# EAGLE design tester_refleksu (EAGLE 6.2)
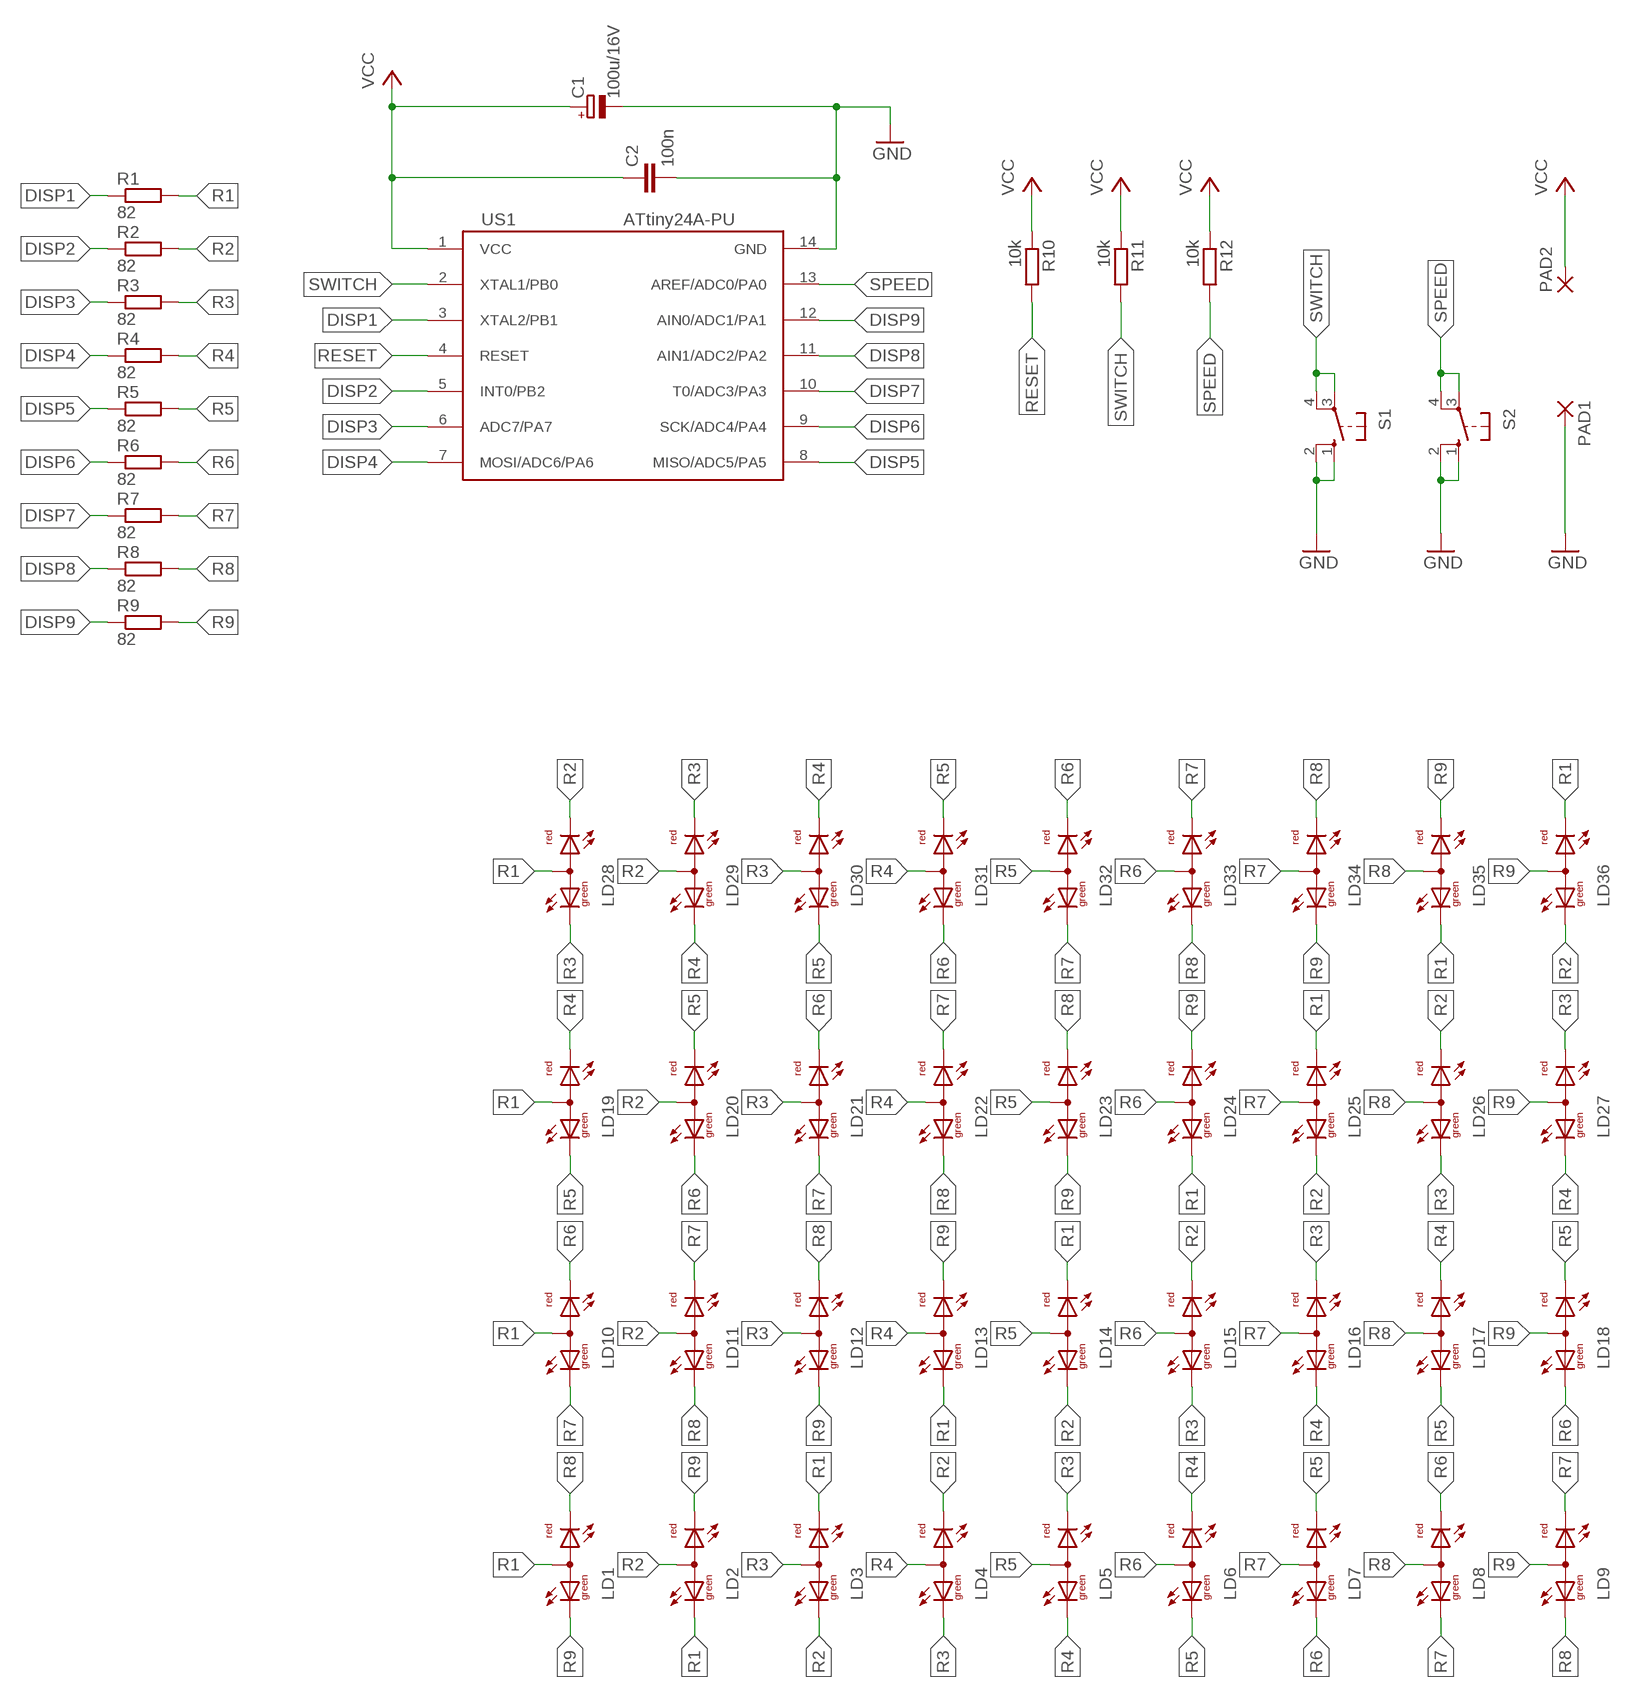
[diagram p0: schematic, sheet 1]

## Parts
C1  100u/16V  CPOL-EUTT2D5L  [TT2D5L]
C2  100n  C-EU050-025X075  [C050-025X075]
LD1  DUOLED-RG-A  [DUOLED-A-5MM]
LD2  DUOLED-RG-A  [DUOLED-A-5MM]
LD3  DUOLED-RG-A  [DUOLED-A-5MM]
LD4  DUOLED-RG-A  [DUOLED-A-5MM]
LD5  DUOLED-RG-A  [DUOLED-A-5MM]
LD6  DUOLED-RG-A  [DUOLED-A-5MM]
LD7  DUOLED-RG-A  [DUOLED-A-5MM]
LD8  DUOLED-RG-A  [DUOLED-A-5MM]
LD9  DUOLED-RG-A  [DUOLED-A-5MM]
LD10  DUOLED-RG-A  [DUOLED-A-5MM]
LD11  DUOLED-RG-A  [DUOLED-A-5MM]
LD12  DUOLED-RG-A  [DUOLED-A-5MM]
LD13  DUOLED-RG-A  [DUOLED-A-5MM]
LD14  DUOLED-RG-A  [DUOLED-A-5MM]
LD15  DUOLED-RG-A  [DUOLED-A-5MM]
LD16  DUOLED-RG-A  [DUOLED-A-5MM]
LD17  DUOLED-RG-A  [DUOLED-A-5MM]
LD18  DUOLED-RG-A  [DUOLED-A-5MM]
LD19  DUOLED-RG-A  [DUOLED-A-5MM]
LD20  DUOLED-RG-A  [DUOLED-A-5MM]
LD21  DUOLED-RG-A  [DUOLED-A-5MM]
LD22  DUOLED-RG-A  [DUOLED-A-5MM]
LD23  DUOLED-RG-A  [DUOLED-A-5MM]
LD24  DUOLED-RG-A  [DUOLED-A-5MM]
LD25  DUOLED-RG-A  [DUOLED-A-5MM]
LD26  DUOLED-RG-A  [DUOLED-A-5MM]
LD27  DUOLED-RG-A  [DUOLED-A-5MM]
LD28  DUOLED-RG-A  [DUOLED-A-5MM]
LD29  DUOLED-RG-A  [DUOLED-A-5MM]
LD30  DUOLED-RG-A  [DUOLED-A-5MM]
LD31  DUOLED-RG-A  [DUOLED-A-5MM]
LD32  DUOLED-RG-A  [DUOLED-A-5MM]
LD33  DUOLED-RG-A  [DUOLED-A-5MM]
LD34  DUOLED-RG-A  [DUOLED-A-5MM]
LD35  DUOLED-RG-A  [DUOLED-A-5MM]
LD36  DUOLED-RG-A  [DUOLED-A-5MM]
PAD1  3,17/1,3  [3,17/1,3]
PAD2  3,17/1,3  [3,17/1,3]
R1  82  R-EU_0207/7  [0207/7]
R2  82  R-EU_0207/7  [0207/7]
R3  82  R-EU_0207/7  [0207/7]
R4  82  R-EU_0207/7  [0207/7]
R5  82  R-EU_0207/7  [0207/7]
R6  82  R-EU_0207/7  [0207/7]
R7  82  R-EU_0207/7  [0207/7]
R8  82  R-EU_0207/7  [0207/7]
R9  82  R-EU_0207/7  [0207/7]
R10  10k  R-EU_0207/7  [0207/7]
R11  10k  R-EU_0207/7  [0207/7]
R12  10k  R-EU_0207/7  [0207/7]
S1  40-XX  [B3F-40XX]
S2  10-XX  [B3F-10XX]
US1  ATtiny24A-PU  ATTINY24/44/84-PU  [DIL14]

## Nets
DISP1: R1.1 US1.3(XTAL2/PB1)
DISP2: R2.1 US1.5(INT0/PB2)
DISP3: R3.1 US1.6(ADC7/PA7)
DISP4: R4.1 US1.7(MOSI/ADC6/PA6)
DISP5: R5.1 US1.8(MISO/ADC5/PA5)
DISP6: R6.1 US1.9(SCK/ADC4/PA4)
DISP7: R7.1 US1.10(T0/ADC3/PA3)
DISP8: R8.1 US1.11(AIN1/ADC2/PA2)
DISP9: R9.1 US1.12(AIN0/ADC1/PA1)
GND: C1.- C2.2 PAD1.1(P) S1.1(S) S1.2(S1) S2.1(S) S2.2(S1) US1.14(GND)
R1: LD1.A LD2.CX(CG) LD3.CR LD10.A LD13.CX(CG) LD14.CR LD19.A LD24.CX(CG) LD25.CR LD28.A LD35.CX(CG) LD36.CR R1.2
R2: LD2.A LD3.CX(CG) LD4.CR LD11.A LD14.CX(CG) LD15.CR LD20.A LD25.CX(CG) LD26.CR LD28.CR LD29.A LD36.CX(CG) R2.2
R3: LD3.A LD4.CX(CG) LD5.CR LD12.A LD15.CX(CG) LD16.CR LD21.A LD26.CX(CG) LD27.CR LD28.CX(CG) LD29.CR LD30.A R3.2
R4: LD4.A LD5.CX(CG) LD6.CR LD13.A LD16.CX(CG) LD17.CR LD19.CR LD22.A LD27.CX(CG) LD29.CX(CG) LD30.CR LD31.A R4.2
R5: LD5.A LD6.CX(CG) LD7.CR LD14.A LD17.CX(CG) LD18.CR LD19.CX(CG) LD20.CR LD23.A LD30.CX(CG) LD31.CR LD32.A R5.2
R6: LD6.A LD7.CX(CG) LD8.CR LD10.CR LD15.A LD18.CX(CG) LD20.CX(CG) LD21.CR LD24.A LD31.CX(CG) LD32.CR LD33.A R6.2
R7: LD7.A LD8.CX(CG) LD9.CR LD10.CX(CG) LD11.CR LD16.A LD21.CX(CG) LD22.CR LD25.A LD32.CX(CG) LD33.CR LD34.A R7.2
R8: LD1.CR LD8.A LD9.CX(CG) LD11.CX(CG) LD12.CR LD17.A LD22.CX(CG) LD23.CR LD26.A LD33.CX(CG) LD34.CR LD35.A R8.2
R9: LD1.CX(CG) LD2.CR LD9.A LD12.CX(CG) LD13.CR LD18.A LD23.CX(CG) LD24.CR LD27.A LD34.CX(CG) LD35.CR LD36.A R9.2
RESET: R10.2 US1.4(RESET)
SPEED: R12.2 S2.3(P) S2.4(P1) US1.13(AREF/ADC0/PA0)
SWITCH: R11.2 S1.3(P) S1.4(P1) US1.2(XTAL1/PB0)
VCC: C1.+ C2.1 PAD2.1(P) R10.1 R11.1 R12.1 US1.1(VCC)

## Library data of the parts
C1 = rcl:CPOL-EU: POLARIZED CAPACITOR, European symbol
C2 = rcl:C-EU: CAPACITOR, European symbol
LD1-LD36 = led:DUOLED-RG-A: DUO LED 2 colors (red/green), 3mm or 5mm, round, common Anode
PAD1 PAD2 = wirepad:3,17/1,3: THROUGH-HOLE PAD
R1-R12 = rcl:R-EU_: RESISTOR, European symbol
S1 = switch-omron:40-XX: OMRON SWITCH; MF: OMRON COMPONENTS USA; MPN: B3F-4000; OC_FARNELL: 176434; OC_NEWARK: 36K3105
S2 = switch-omron:10-XX: OMRON SWITCH; MPN: B3F-1000; OC_FARNELL: 176432; OC_NEWARK: 36M3542
US1 = scalaki_futrzak:ATTINY24/44/84

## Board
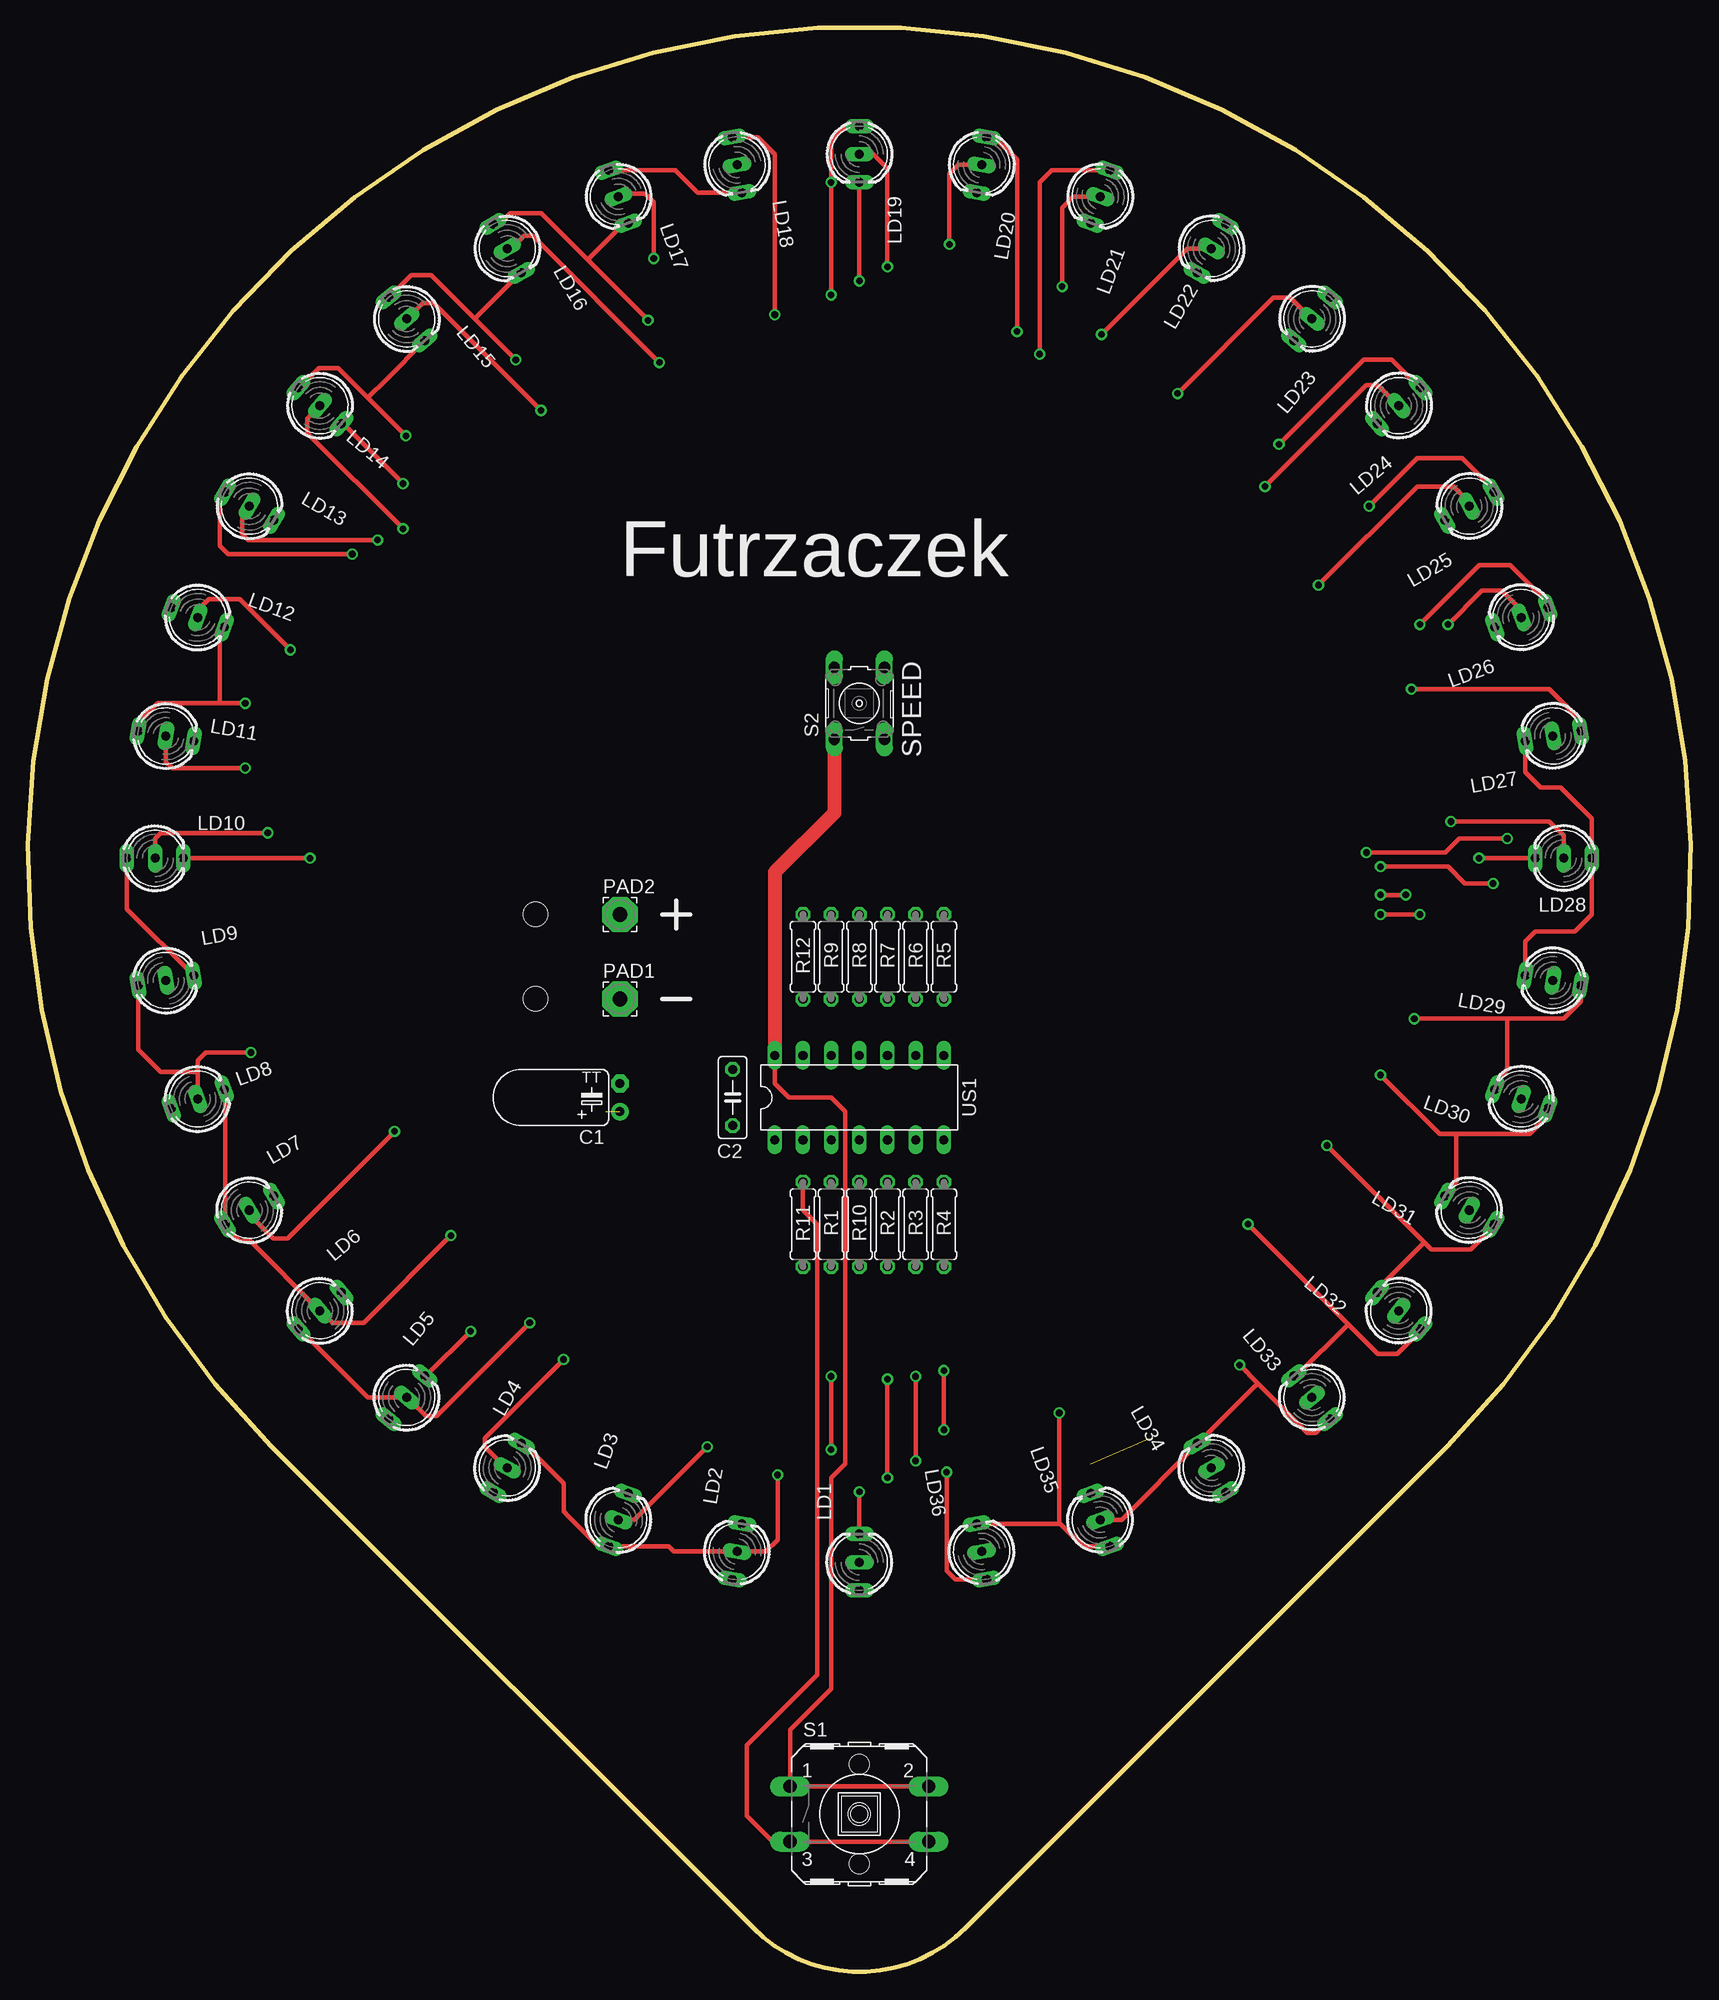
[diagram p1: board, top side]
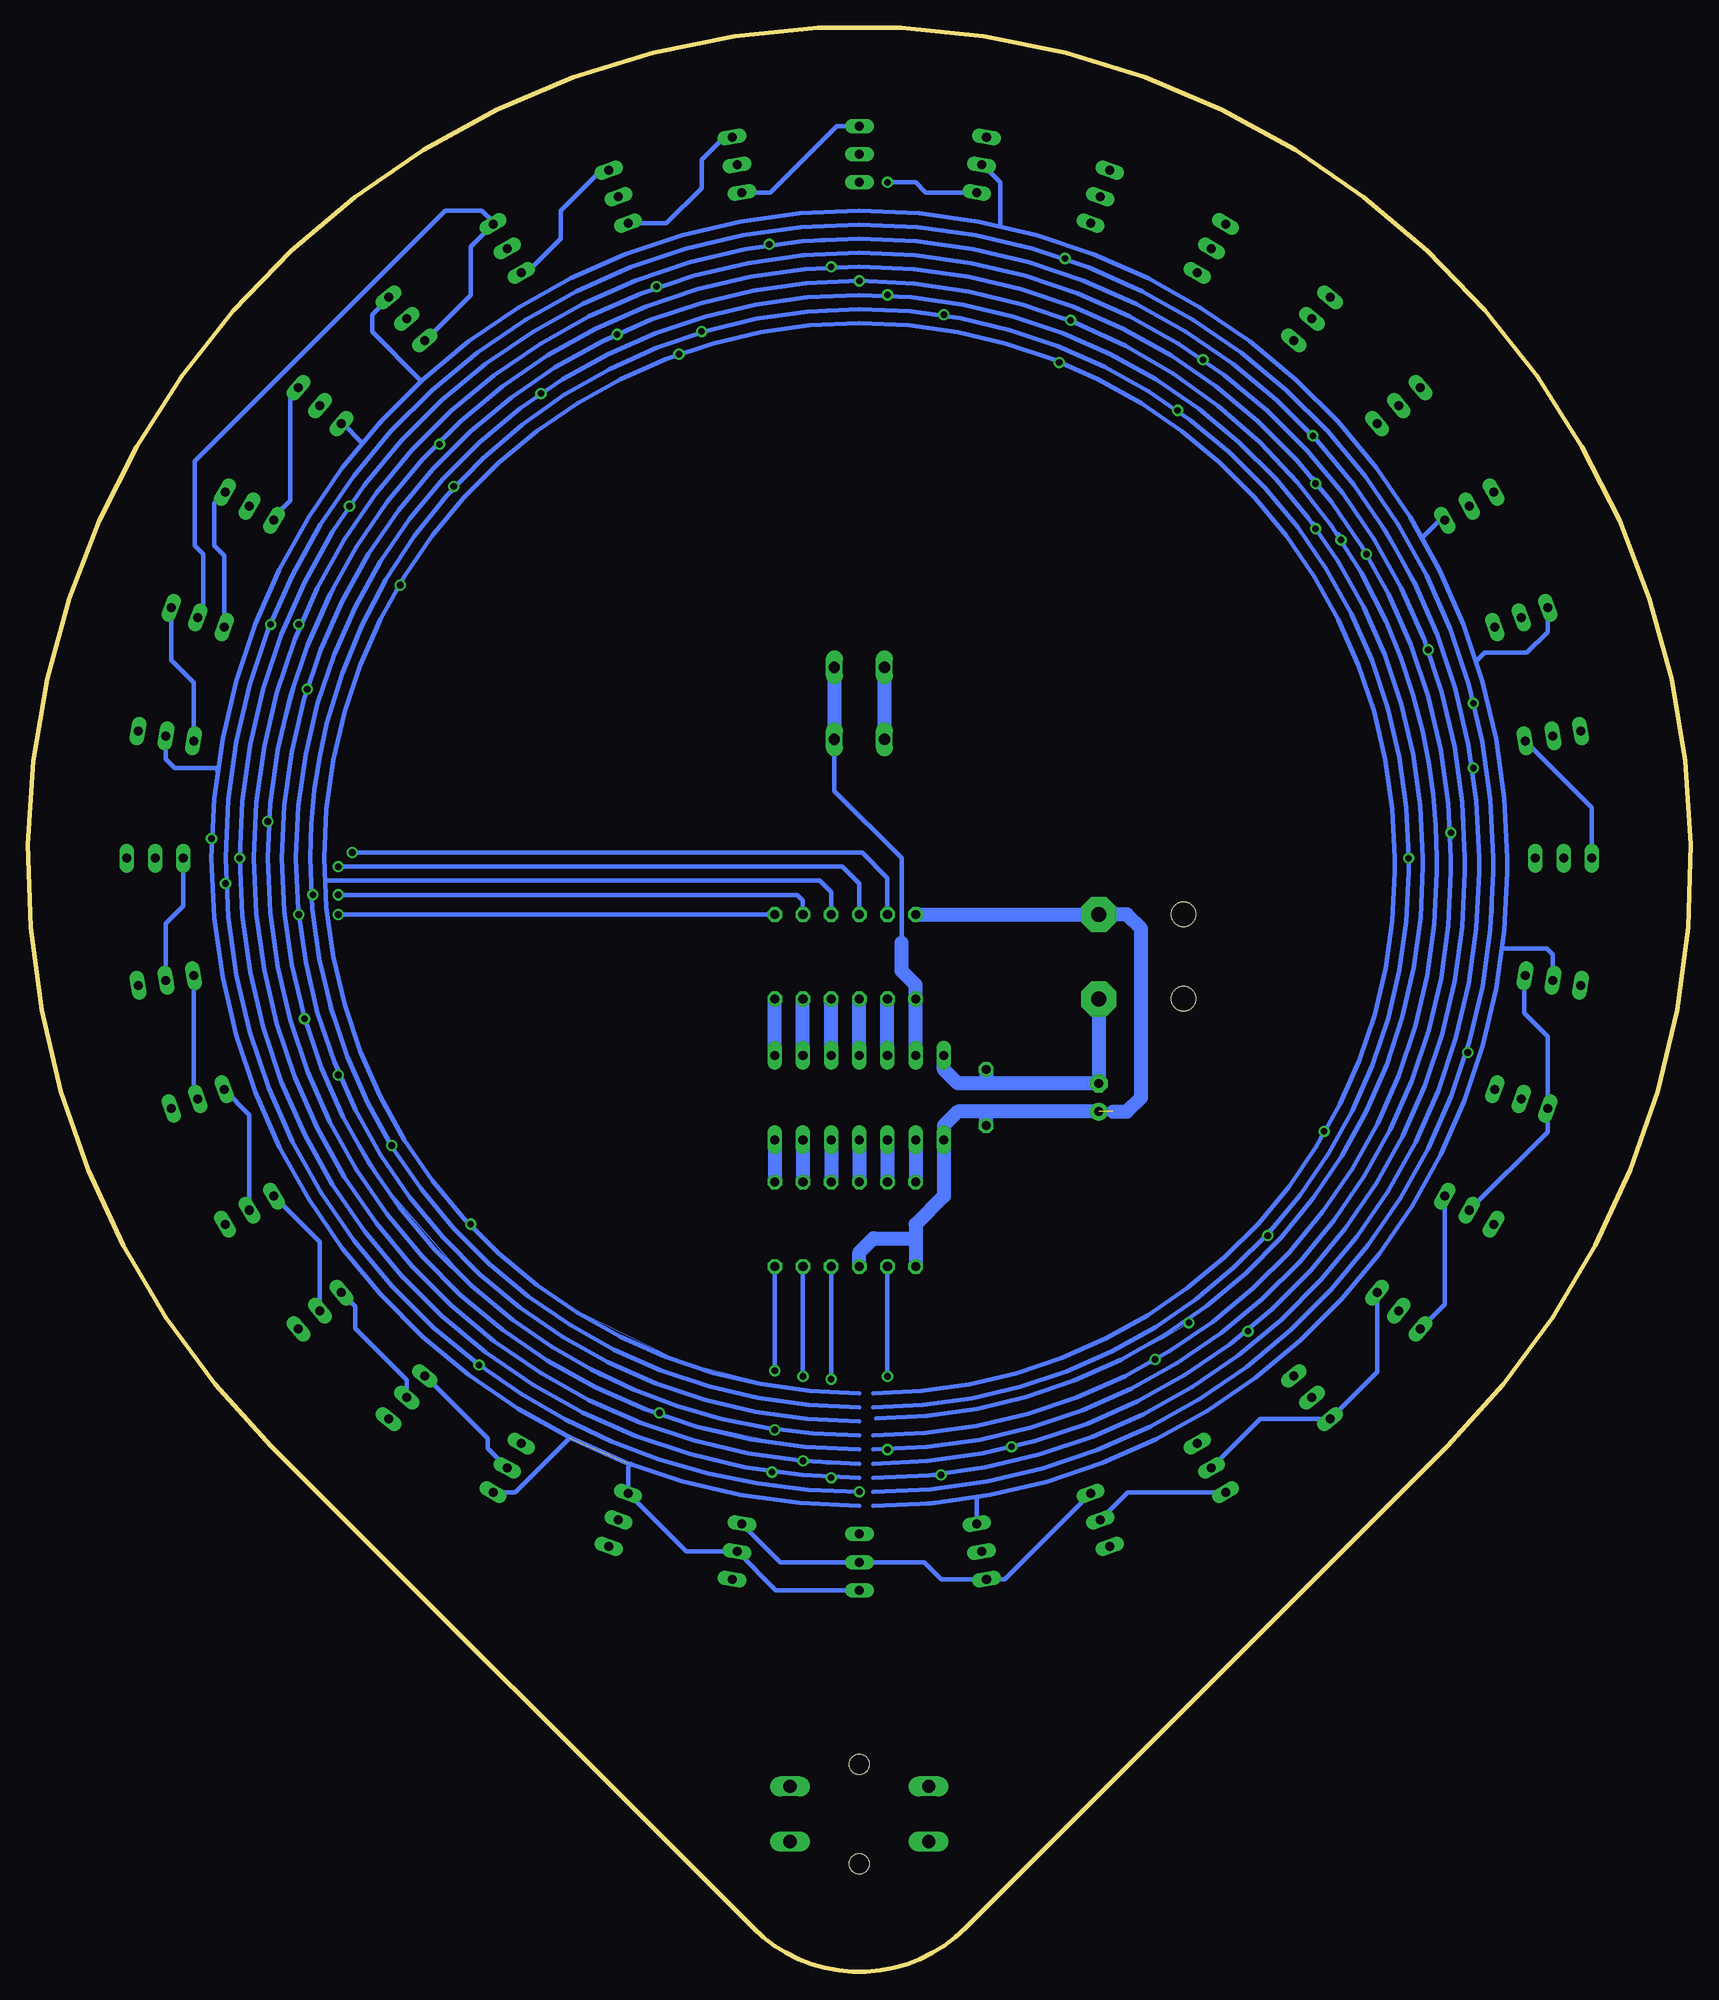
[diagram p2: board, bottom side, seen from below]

Size 149.98 x 175.35 mm. Coordinates in mm from the lower left corner, seen from the top.
Outline: 21.96,47.41 65.42,3.95 arc90 84.56,3.95 128.02,47.41 arc270 21.96,47.41
Copper layers (1*16): Top 0.035mm / dielectric 1.5mm / Bottom 0.035mm
Design rules: minimum track width 10mil, minimum drill 23mil, track to track 8mil, track to pad 8mil, pad to pad 8mil, via to via 8mil, smd to smd 8mil, copper to edge 15mil, drill to drill 8mil, minimum pad ring 10mil, minimum via ring 8mil, stop-mask expansion 4mil, vias tented up to drill 0mil, thermal gap 10mil
Holes 2.2 mm at 45.78,87.74 45.78,95.36

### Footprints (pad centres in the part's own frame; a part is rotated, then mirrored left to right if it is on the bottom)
TT2D5L = drill 0.813 pad 1.6: + -1.27,0 | drill 0.813 pad 1.6 octagon: - 1.27,0
C050-025X075 = drill 0.813 octagon: 1 -2.54,0; 2 2.54,0
DUOLED-A-5MM = drill 0.813 long: A 0,0; CR 2.54,0; CX -2.54,0
3,17/1,3 = drill 1.321 pad 3.175 octagon: 1 0,0
0207/7 = drill 0.813 octagon: 1 -3.81,0; 2 3.81,0
B3F-40XX = drill 1.194 long: 1 -6.248,2.489; 2 6.248,2.489; 3 -6.248,-2.489; 4 6.248,-2.489 | hole 1.803: 0,-4.496; 0,4.496
B3F-10XX = drill 1.016 long: 1 -3.251,2.261; 2 3.251,2.261; 3 -3.251,-2.261; 4 3.251,-2.261
DIL14 = drill 0.813 long: 1 -7.62,-3.81; 2 -5.08,-3.81; 3 -2.54,-3.81; 4 0,-3.81; 5 2.54,-3.81; 6 5.08,-3.81; 7 7.62,-3.81; 8 7.62,3.81; 9 5.08,3.81; 10 2.54,3.81; 11 0,3.81; 12 -2.54,3.81; 13 -5.08,3.81; 14 -7.62,3.81

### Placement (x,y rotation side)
C1  53.4,78.85 90 top
C2  63.56,78.85 90 top
LD1  74.99,36.94 90 top
LD2  63.96,37.91 80 top
LD3  53.27,40.77 70 top
LD4  43.24,45.45 60 top
LD5  34.17,51.8 50 top
LD6  26.35,59.63 40 top
LD7  20,68.69 30 top
LD8  15.32,78.72 20 top
LD9  12.45,89.42 10 top
LD10  11.49,100.44 0 top
LD11  12.45,111.47 350 top
LD12  15.32,122.16 340 top
LD13  20,132.19 330 top
LD14  26.35,141.26 320 top
LD15  34.17,149.09 310 top
LD16  43.24,155.44 300 top
LD17  53.27,160.11 290 top
LD18  63.96,162.98 280 top
LD19  74.99,163.94 270 top
LD20  86.02,162.98 260 top
LD21  96.71,160.11 250 top
LD22  106.74,155.44 240 top
LD23  115.81,149.09 230 top
LD24  123.63,141.26 220 top
LD25  129.98,132.19 210 top
LD26  134.66,122.16 200 top
LD27  137.52,111.47 190 top
LD28  138.49,100.44 180 top
LD29  137.52,89.42 170 top
LD30  134.66,78.72 160 top
LD31  129.98,68.69 150 top
LD32  123.63,59.63 140 top
LD33  115.81,51.8 130 top
LD34  106.74,45.45 120 top
LD35  96.71,40.77 110 top
LD36  86.02,37.91 100 top
PAD1  53.4,87.74 0 top
PAD2  53.4,95.36 0 top
R1  72.45,67.42 270 top
R2  77.53,67.42 270 top
R3  80.07,67.42 270 top
R4  82.61,67.42 270 top
R5  82.61,91.55 90 top
R6  80.07,91.55 90 top
R7  77.53,91.55 90 top
R8  74.99,91.55 90 top
R9  72.45,91.55 90 top
R10  74.99,67.42 90 top
R11  69.91,67.42 90 top
R12  69.91,91.55 270 top
S1  74.99,14.23 0 top
S2  74.99,114.41 90 top
US1  74.99,78.85 0 top

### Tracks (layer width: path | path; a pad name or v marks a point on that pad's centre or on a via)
DISP1
  Bottom 1.27: US1.3 R1.1
DISP2
  Bottom 1.27: US1.5 R2.1
DISP3
  Bottom 1.27: US1.6 R3.1
DISP4
  Bottom 1.27: US1.7 R4.1
DISP5
  Bottom 1.27: US1.8 R5.1
DISP6
  Bottom 1.27: US1.9 R6.1
DISP7
  Bottom 1.27: US1.10 R7.1
DISP8
  Bottom 1.27: US1.11 R8.1
DISP9
  Bottom 1.27: US1.12 R9.1
GND
  Top 0.406: S1.2 S1.1 68.74,21.81 72.45,25.51 72.45,44.56 73.72,45.83 73.72,77.58 72.45,78.85 68.64,78.85 67.37,80.12 US1.14
  Top 1.27: S2.1 72.73,104.53 67.37,99.17 US1.14
  Bottom 1.27: 63.56,80.12 C1.- PAD1.1 | 63.56,80.12 66.1,80.12 67.37,81.39 US1.14 | C2.2 63.56,80.12 | S2.2 S2.1
R1  (via drill 0.6)
  Top 0.406: LD19.A 76.26,163.94 77.53,162.67 v77.53,153.78 | LD24.CX 125.5,142.89 123,145.4 120.46,145.4 v112.84,137.78 | LD28.A 138.49,102.48 137.22,103.75 v128.33,103.75 | LD35.CX 95.14,38.39 94.29,39.23 93.02,40.5 | 93.02,40.5 v93.02,50.41 | LD36.CR 92.93,40.41 93.02,40.5 | LD10.A 11.49,102.22 12,102.73 v21.65,102.73 | LD13.CX 17.8,133.17 17.33,132.7 17.33,128.64 18.09,127.88 v29.27,127.88 | LD14.CR 28.44,139.63 v33.84,134.23 | v72.45,53.71 v72.45,47.1
  Bottom 0: 128.33,100.44 v128.33,103.75 128.08,106.03 127.57,109.33 125.28,117.97 120.96,127.62 115.63,134.99 v112.84,137.78 | 74.99,47.1 78.55,47.1 83.12,47.87 89.98,49.39 v93.02,50.41 | 73.72,47.1 v72.45,47.1 | 21.65,100.44 v21.65,102.73 21.9,106.29 22.41,109.08 22.67,111.37 24.19,116.95 24.95,118.99 25.97,121.27 26.73,123.3 v29.27,127.88 | 29.52,128.13 33.08,133.46 v33.84,134.23 | v77.53,153.78 74.99,153.78
  Bottom 0.406: 74.99,47.1 arc90 128.33,100.44 arc90 74.99,153.78 arc90 21.65,100.44 21.65,99.17 arc90 73.72,47.1 | LD25.CR 127.78,131.22 126.3,132.7 126.3,142.17 LD24.CX | LD36.CR 82.11,36.94 LD1.A 69.15,36.94 67.61,35.41 LD2.CX 61.89,35.41 LD3.CR | v21.65,102.73 21.65,102.22 | v29.27,127.88 29.52,128.13 | v33.84,134.23 33.84,134.48 34.1,134.73 | R1.2 v72.45,53.71 | v72.45,47.1 72.2,47.1
R2  (via drill 0.6)
  Top 0.406: LD20.A 83.93,162.98 83.12,162.17 v83.12,155.82 | LD25.CX 132.18,133.68 129.35,136.51 125.28,136.51 v120.96,132.19 | LD28.CR v130.87,100.44 | LD36.CX 83.64,35.41 82.86,36.18 v82.86,45.07 | v67.62,44.82 67.62,38.98 66.56,37.91 LD2.A 58.28,37.91 57.97,38.21 57.8,38.39 LD3.CX 51.45,38.39 48.83,41.01 48.32,41.52 48.32,44.06 44.72,47.65 LD4.CR | LD11.A 12.45,109.13 13.01,108.57 v19.62,108.57 | LD14.CX 24.48,142.89 26.22,144.64 28,144.64 30.67,141.97 | 30.67,141.97 v34.1,138.54 | LD15.CR 35.81,147.11 32.32,143.62 30.67,141.97 | v77.53,53.45 v77.53,44.56
  Bottom 0: v130.87,100.44 130.36,107.3 129.35,113.14 128.58,116.19 127.31,120.26 126.04,123.3 124.01,127.37 v120.96,132.19 | 77.28,44.56 74.99,44.56 | v82.86,45.07 79.31,44.82 v77.53,44.56 | 68.39,44.82 71.18,44.56 73.72,44.56 | 19.11,100.44 19.36,104.76 v19.62,108.57 | 19.87,109.08 20.38,112.89 23.43,122.03 26.48,127.88 28.76,131.69 31.3,135.24 v34.1,138.54 | 74.99,156.32 78.55,156.32 81.34,156.07 v83.12,155.82
  Bottom 0.406: 74.99,44.56 arc90 v130.87,100.44 arc90 74.99,156.32 arc90 19.11,100.44 19.11,99.17 arc90 73.72,44.56 | LD26.CR 132.27,127.76 133.16,128.64 133.16,132.49 LD25.CX | LD28.CR 135.95,96.13 137.52,94.55 LD29.A | v67.62,44.82 68.39,44.82 | v19.62,108.57 19.62,108.83 19.87,109.08 | v34.1,138.54 34.35,138.8 | R2.2 v77.53,53.45 | v77.53,44.56 77.28,44.56
R3  (via drill 0.6)
  Top 0.406: LD21.A 94.27,160.11 93.28,159.12 v93.28,152.01 | LD26.CX 137.05,123.48 133.66,126.86 130.87,126.86 v125.54,121.53 | LD27.CR 135.02,108.23 136.46,106.79 138.24,106.79 141.03,104 LD28.CX 141.03,95.36 139.51,93.84 135.95,93.84 135.02,92.91 LD29.CR | LD3.A 54.69,40.77 v61.27,47.36 | LD5.CR 35.91,53.75 v39.94,57.77 | LD12.A 15.32,122.82 16.32,123.81 19.11,123.81 v23.68,119.24 | LD15.CX 32.62,151.03 34.6,153.02 36.38,153.02 40.32,149.08 | 40.32,149.08 v44,145.4 | LD16.CR 44.47,153.24 40.32,149.08 | v80.07,53.71 v80.07,46.09
  Bottom 0: 129.6,100.44 129.35,105.78 128.58,110.86 126.3,118.99 v125.54,121.53 | 79.82,46.09 78.04,45.83 74.99,45.83 | 73.72,45.83 71.69,45.83 67.37,46.34 62.54,47.1 v61.27,47.36 59.75,47.61 53.15,49.9 47.05,52.95 43.24,55.49 v39.94,57.77 | 20.38,104 20.89,108.57 21.9,112.89 22.67,115.94 v23.68,119.24 22.41,115.18 21.14,110.1 20.38,104 | v93.28,152.01 89.98,153.02 83.88,154.29 79.05,154.8 76.51,155.05 74.99,155.05 73.21,155.05 70.16,154.8 64.32,154.04 60.26,153.02 54.16,150.99 49.59,148.7 45.53,146.42 v44,145.4 | 20.38,104 20.38,100.44
  Bottom 0.406: 74.99,45.83 arc90 129.6,100.44 arc90 74.99,155.05 arc90 20.38,100.44 20.38,99.17 arc90 73.72,45.83 | LD27.CR 135.02,116.28 137.05,118.3 LD26.CX | LD29.CR 135.02,79.09 LD30.A | LD4.CX 50.79,43.25 LD3.A | v23.68,119.24 23.94,119.49 | R3.2 v80.07,53.71 | v80.07,46.09 79.82,46.09
R4  (via drill 0.6)
  Top 0.406: LD19.CR v74.99,152.51 | LD22.A 104.58,155.44 v96.83,147.69 | LD27.CX 140.03,112.88 137.22,115.68 v124.77,115.68 | LD29.CX 140.03,87.5 138.49,85.97 133.41,85.97 | 133.41,85.97 v125.03,85.97 | LD30.CR 132.27,80.26 133.41,81.39 133.41,85.97 | LD4.A 43.11,45.45 41.21,47.36 41.21,48.12 v48.32,55.23 | LD13.A 20,132.06 19.36,131.43 19.36,129.65 19.87,129.15 v31.56,129.15 | LD16.CX 42.52,157.64 43.49,158.61 46.29,158.61 50.48,154.42 | 50.48,154.42 v55.94,148.96 | LD17.CR 53.79,157.73 50.48,154.42 | v82.61,54.22 v82.61,48.88
  Bottom 0: v124.77,115.68 125.54,113.14 126.3,109.33 127.06,102.73 127.06,100.44 127.06,97.14 126.3,92.06 125.54,88.25 v125.03,85.97 124.52,84.95 122.23,78.35 117.66,70.73 110.55,62.6 106.23,58.79 102.17,55.99 98.36,53.71 95.31,52.44 91.5,50.91 85.66,49.39 v82.61,48.88 | 73.72,48.37 66.1,48.88 57.21,51.17 51.11,53.71 v48.32,55.23 | 22.92,100.44 22.92,102.73 23.17,105.78 23.68,108.57 24.19,111.87 25.21,115.43 26.48,119.24 27.49,121.78 29.27,125.08 30.03,126.86 v31.56,129.15 | 56.19,148.96 59.24,149.97 66.35,151.75 70.42,152.26 v74.99,152.51 79.05,152.26 84.9,151.5 89.21,150.48 95.31,148.45 v96.83,147.69
  Bottom 0.406: 74.99,48.37 arc37 106.23,58.79 arc53 127.06,100.44 arc90 v74.99,152.51 arc66 27.49,121.78 arc12 24.19,111.87 arc13 22.92,100.44 22.92,99.17 arc90 73.72,48.37 | LD31.A 129.98,77.3 LD30.CR | v48.32,55.23 48.57,54.98 | LD4.A 38.84,49.85 LD5.CX 28.29,54.1 LD6.CR | v31.56,129.15 31.56,129.4 31.81,129.65 | v55.94,148.96 56.19,148.96 | R4.2 v82.61,54.22 | v82.61,48.88 82.86,48.88
R5  (via drill 0.6)
  Top 0.406: LD19.CX 73.72,166.48 72.45,165.21 v72.45,161.4 v72.45,151.24 | LD23.A 115.75,149.09 113.85,150.99 112.33,150.99 v103.69,142.35 | LD30.CX 137.05,77.16 135.44,75.55 128.84,75.55 | 128.84,75.55 127.31,75.55 v121.98,80.89 | LD31.CR 127.78,70.18 128.84,71.23 128.84,75.55 | v45.27,58.53 36.89,50.15 35.87,50.15 34.23,51.8 LD5.A 30.67,51.8 24.48,57.99 LD6.CX | LD14.A 26.35,141.21 25.21,140.07 25.21,138.8 v33.84,130.16 | LD17.CX 58.4,162.5 60.42,160.48 LD18.CR | v121.98,95.36 v125.54,95.36
  Bottom 0: 125.54,95.87 125.79,97.9 125.79,100.44 | v121.98,80.89 123.76,85.97 125.28,92.82 v125.54,95.36 | v45.27,58.53 47.81,57.01 52.13,54.72 55.69,53.2 63.81,50.91 70.16,50.15 73.47,49.9 | 24.19,100.44 24.44,104.25 24.95,109.08 25.71,112.64 26.22,114.92 27.49,118.73 29.02,122.03 29.78,123.3 31.3,126.35 v33.84,130.16 | v72.45,151.24 74.99,151.24 77.02,151.24 82.61,150.74 87.69,149.72 90.74,148.7 96.33,146.67 99.12,145.15 101.66,143.62 v103.69,142.35
  Bottom 0.406: 74.99,49.64 arc90 125.79,100.44 arc90 74.99,151.24 arc90 24.19,100.44 24.19,99.68 arc90 73.47,49.9 | LD18.CR 68.98,160.48 69.91,161.4 v72.45,161.4 | LD20.CR 83.03,160.48 77.02,166.48 LD19.CX | LD19.CX | LD32.A 123.63,65.81 LD31.CR | LD7.CR 22.2,60.2 LD6.CX | v33.84,130.16 33.84,130.42 34.1,130.67 | R5.2 v121.98,95.36 | v125.54,95.36 125.54,95.87
R6  (via drill 0.6)
  Top 0.406: LD18.CX 65.83,165.48 67.37,163.94 v67.37,149.47 | LD20.CX 87.17,165.48 89.21,163.44 v89.21,147.94 | LD24.A 123.58,141.26 121.73,143.12 120.71,143.12 v111.57,133.97 | LD31.CX 132.18,67.21 130.11,65.14 126.55,65.14 125.92,65.77 | 125.92,65.77 v117.15,74.54 | LD32.CR 121.69,61.54 125.92,65.77 | v38.16,66.41 30.29,58.53 27.49,58.53 26.4,59.63 LD6.A 20.07,65.9 19.11,65.9 17.8,67.21 LD7.CX 17.8,79.5 LD8.CR | LD10.CR v25.46,100.44 | LD15.A 34.23,149.09 35.62,150.48 36.64,150.48 v46.29,140.83 | v121.98,97.14 v124.27,97.14
  Bottom 0: 124.52,97.14 124.51,99.13 124.52,100.44 124.27,105.78 123,112.64 120.71,119.75 118.93,123.05 116.9,126.86 115.12,129.65 113.34,131.69 v111.57,133.97 | v117.15,74.54 119.19,77.84 120.96,82.16 122.74,86.73 124.01,93.08 v124.27,97.14 | v25.46,100.44 25.97,92.32 27.24,85.97 28.76,81.65 31.56,75.81 33.84,72 36.38,68.69 v38.16,66.41 | v67.37,149.47 71.94,149.97 73.47,149.97 | v67.37,149.47 69.91,149.72 73.47,149.97 | 73.47,149.97 74.99,149.97 76.26,149.97 | 76.26,149.97 79.82,149.72 84.13,149.21 v89.21,147.94 87.69,148.2 83.12,149.21 78.04,149.97 76.26,149.97 | v46.29,140.83 48.32,142.1 51.11,143.88 54.16,145.4 57.46,146.67 61.02,147.94 64.58,148.96 v67.37,149.47
  Bottom 0.406: 74.99,50.91 arc90 124.52,100.44 arc14 123,112.64 arc76 74.99,149.97 arc90 v25.46,100.44 25.46,99.17 arc90 73.72,50.91 | LD21.CR 92.38,157.73 89.21,160.9 89.21,163.44 87.17,165.48 LD20.CX | LD33.A 115.81,53.38 120.46,58.03 120.46,60.03 LD32.CR | v38.16,66.41 38.16,66.66 37.91,66.92 | v46.29,140.83 46.03,140.58 | R6.2 80.07,96.63 80.58,97.14 v121.98,97.14 | v124.27,97.14 124.52,97.14
R7  (via drill 0.6)
  Top 0.406: LD21.CX 92.34,162.5 91.25,161.4 v91.25,145.91 | LD25.A 129.98,132.57 128.58,133.97 125.28,133.97 v116.39,125.08 | LD32.CX 125.58,57.82 123.5,55.74 121.73,55.74 119.06,58.41 | 119.06,58.41 v110.04,67.42 | LD33.CR 114.4,53.75 119.06,58.41 | LD7.A 20,68.31 22.16,66.15 23.43,66.15 v33.08,75.81 | LD10.CX 8.95,95.86 LD9.CR | LD16.A 43.62,155.44 44.76,156.58 45.53,156.58 v56.96,145.15
  Bottom 0: 123,98.41 123.25,98.41 | 123.25,98.41 123.25,100.44 123,105.78 121.98,111.11 119.95,117.72 117.15,123.81 v116.39,125.08 | 74.99,52.18 76.01,52.18 82.1,52.69 90.99,54.98 101.41,60.06 | v110.04,67.42 111.57,68.95 113.85,71.74 117.15,76.82 119.69,82.66 121.22,86.98 122.23,90.28 123,94.6 123.25,98.41 | 26.73,99.17 26.98,94.35 27.75,90.28 28,88 29.52,83.17 31.81,78.09 v33.08,75.81 | v56.96,145.15 59.24,146.16 63.31,147.18 66.86,147.94 70.67,148.45 74.99,148.7 79.31,148.45 83.88,147.94 86.67,147.18 v91.25,145.91
  Bottom 0.406: 74.99,52.18 arc90 123.25,100.44 arc90 74.99,148.7 arc90 26.73,100.44 26.73,99.17 arc90 73.72,52.18 | LD21.CX 98.28,162.5 101.91,158.86 101.91,156.32 105,153.24 LD22.CR | LD33.CR 114.14,53.75 108.52,48.12 108.52,47.23 LD34.A | v33.08,75.81 33.08,75.55 33.33,75.3 | LD7.A 12.93,75.76 LD8.CX 12.93,84.36 15.05,86.47 15.05,89.77 LD9.CR | LD10.CX 8.95,105.02 LD11.CR | v56.96,145.15 56.7,145.15 | R7.2 77.53,97.4 78.55,98.41 123,98.41
R8  (via drill 0.6)
  Top 0.406: LD26.A 134.66,122.82 132.9,124.57 131.12,124.57 v128.08,121.53 | LD33.CX 117.36,49.85 116.14,48.63 115.38,48.63 110.93,53.07 | 110.93,53.07 v109.28,54.72 | 110.93,53.07 105.51,47.65 LD34.CR 105.47,47.61 98.63,40.77 LD35.A | LD1.CR v74.99,43.29 | LD8.A 15.32,81.14 | 15.32,81.14 15.32,82.18 16.06,82.92 v20.13,82.92 | LD9.CX 9.95,83.18 12,81.14 15.32,81.14 | LD11.CX 9.95,112.62 11.74,114.41 17.33,114.41 | 17.33,114.41 v19.62,114.41 | LD12.CR 17.71,120.63 17.33,120.26 17.33,114.41 | LD17.A 53.89,160.11 54.16,160.39 55.69,160.39 56.45,159.63 v56.45,154.55 | v121.98,99.68 128.08,99.68 129.6,98.16 v132.14,98.16
  Bottom 0: 132.14,98.41 132.14,100.44 132.14,102.48 131.63,107.3 131.12,110.86 129.85,115.94 v128.08,121.53 | 17.84,99.17 17.84,95.62 18.35,91.81 19.36,86.47 20.13,83.43 v20.13,82.92 | 17.84,100.44 18.09,104.76 18.6,108.83 19.11,112.13 v19.62,114.41 | v56.45,154.55 57.46,154.8 61.02,155.82 65.59,156.83 70.42,157.34 74.99,157.59 78.04,157.59 82.1,157.09 86.93,156.32 90.23,155.56 92.77,154.8 98.1,152.77 102.42,150.48 105.47,148.7
  Bottom 0.406: v74.99,43.29 arc37 v109.28,54.72 arc53 132.14,100.44 arc90 74.99,157.59 arc90 17.84,100.44 17.84,99.17 arc90 73.72,43.29 | LD23.CR 114.14,147.14 110.04,151.24 110.04,155.6 LD22.CX 108.01,157.85 109.03,158.86 112.33,158.86 134.93,136.26 134.93,128.64 134.17,127.88 134.17,122.65 LD26.A | v20.13,82.92 20.38,82.66 | v19.62,114.41 19.62,114.16 | v56.45,154.55 56.19,154.29 | R8.2 74.99,98.16 76.51,99.68 v121.98,99.68 | v132.14,98.16 132.14,98.41
R9  (via drill 0.6)  (1 unrouted)
  Top 0.406: v120.71,100.95 127.82,100.95 129.09,102.22 v133.41,102.22
  Bottom 0: 133.41,100.44 v133.41,102.22 133.41,102.98 133.16,105.78 132.9,108.32 | 95.84,45.56 95.82,45.83 92.01,44.56 84.64,42.79 78.8,42.28 74.99,42.02 | 64.32,42.79 69.91,42.28 73.72,42.02 | 16.82,92.32 17.08,92.32 16.82,95.36 16.57,99.17 | 16.57,100.44 16.82,105.52 17.59,111.37 18.6,115.18 19.36,118.22 20.63,121.53 22.67,126.35 24.19,129.4 | 62.29,157.59 64.83,157.85 68.89,158.61 71.94,158.86 74.99,158.86 76.77,158.86 | 114.61,143.62 114.36,143.62 111.82,145.91 108.77,148.2 106.49,149.72 103.95,151.24 100.14,153.28 97.85,154.29 92.52,156.07 87.69,157.59 84.9,158.1 80.83,158.61 76.77,158.86 | 114.61,143.62 112.84,144.89 109.28,147.69 105.47,150.23 102.17,152.26 98.87,153.78 94.29,155.56 90.23,156.83 85.91,157.85 84.13,158.1 79.82,158.61 78.55,158.86 76.77,158.86 | 119.95,138.04 119.95,137.78 121.47,135.75 115.88,142.1 114.61,143.62
  Bottom 0.406: 74.99,42.02 arc90 133.41,100.44 arc90 74.99,158.86 arc90 16.57,100.44 16.57,99.17 arc90 73.72,42.02 | LD18.A 63.86,162.98 62.29,161.4 62.29,157.59 | LD23.CX 117.44,150.96 118.93,149.47 118.93,147.94 114.61,143.62 | LD24.CR 121.54,139.63 119.95,138.04 | LD27.A 137.52,109.38 136.71,108.57 132.9,108.57 132.9,108.32 | LD34.CX 106.02,43.25 101.15,48.12 | 95.56,45.83 95.84,45.56 LD35.CR 90.59,37.91 LD36.A 82.51,34.4 LD1.CX | LD2.CR 64.4,42.7 64.32,42.79 | LD9.A 12.45,91.76 13.01,92.32 16.82,92.32 | LD12.CX 12.93,120.84 14.79,118.99 18.6,118.99 19.36,118.22 | LD13.CR 22.67,130.92 24.19,129.4 | R9.2 72.45,98.67 74.74,100.95 v120.71,100.95 | 133.41,102.48 v133.41,102.22 133.41,101.97
RESET
  Bottom 1.27: US1.4 R10.2
SPEED
  Bottom 0.406: 71.18,92.82 71.18,100.44 77.25,106.51 S2.3
  Bottom 1.27: US1.13 R12.2 69.91,89.01 71.18,90.28 71.18,92.82 | S2.4 S2.3
SWITCH
  Top 0.406: R11.2 69.91,68.69 71.18,67.42 71.18,26.78 64.83,20.43 64.83,14.08 67.17,11.74 S1.3 S1.4
  Bottom 1.27: US1.2 R11.2
VCC  (1 unrouted)
  Bottom 1.27: C1.+ 63.56,77.58 | 63.56,77.58 66.1,77.58 67.37,76.31 US1.1 67.37,69.96 69.91,67.42 69.91,66.15 | C2.1 63.56,77.58 | R12.1 PAD2.1 50.86,95.36 49.59,94.09 49.59,78.85 50.86,77.58 52.13,77.58 | 69.91,66.15 R11.1 | R10.1 74.99,64.88 73.72,66.15 69.91,66.15

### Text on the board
tPlace: Futrzaczek | SPEED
